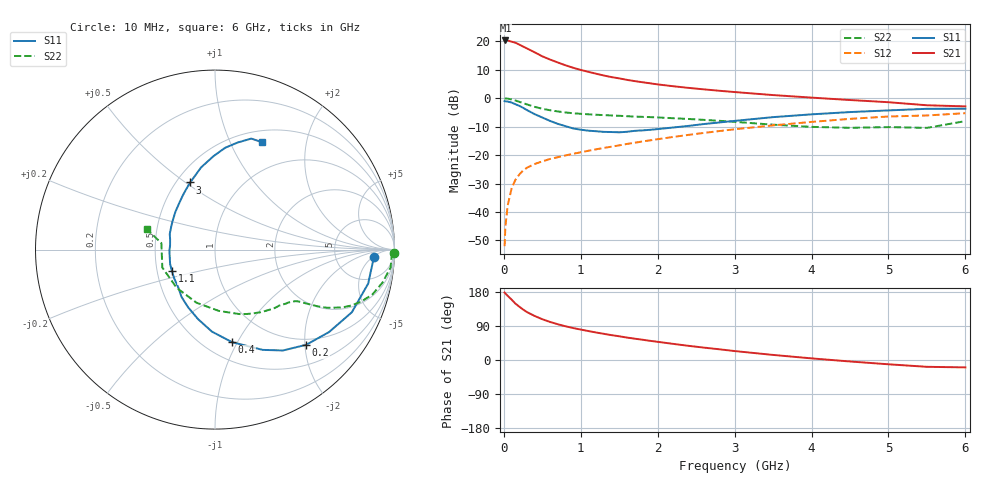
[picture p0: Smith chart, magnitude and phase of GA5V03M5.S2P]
! Infineon Technologies  Discrete & RF Semiconductors
! BF775
! Si NPN RF Bipolar Junction Transistor in SOT23
! VCE = 5 V  IC = 3.5 mA
! Common Emitter S-Parameters:  May  1996
# GHz  S  MA  R  50
!  f  S11  S21  S12  S22
! GHz  MAG  ANG  MAG  ANG  MAG  ANG  MAG  ANG
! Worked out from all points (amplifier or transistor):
!   36 points, 10 MHz to 6 GHz, reference 50 ohm
!   highest |S21| = 20.3 dB at 20 MHz (marker M1)
!   |S21| within 3 dB of that: start of sweep to 315.4 MHz
!   unconditionally stable (mu >= 1): 945.7 MHz to 3.352 GHz
!   at 250 MHz: K = 0.38, MSG = 21.8 dB, |S12| = -25.4 dB
!   at 1.4 GHz: K = 1.12, MAG = 10.2 dB, |S12| = -17.0 dB
!   at 6 GHz: K = 0.95, MSG = 1.2 dB, |S12| = -5.3 dB
!   S11 on the Smith chart (normalised r, x): 10 MHz: 15, -5; 200 MHz: 0.88, -2.03; 400 MHz: 0.67, -0.95; 1.1 GHz: 0.60, -0.15; 3 GHz: 0.59, +0.52; 6 GHz: 0.64, +1.33
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0.01  0.8876 -2.5  10.25 177.9  0.0025 86.6  0.9951 -1.1
0.02  0.8812 -5.0  10.36 175.5  0.0055 85.3  0.9848 -2.2
0.05  0.8742 -12.5  10.33 169.3  0.013 84.0  0.9832 -5.8
0.1  0.8386 -24.6  9.869 159.5  0.0256 76.8  0.9516 -11.1
0.15  0.784 -35.9  9.449 148.9  0.0366 70.3  0.9121 -15.9
0.2  0.7345 -46.2  8.785 140.9  0.0454 66.2  0.8656 -19.5
0.25  0.6779 -56.0  8.1 133.3  0.0534 62.2  0.8209 -22.3
0.3  0.6185 -64.6  7.516 126.5  0.0599 59.9  0.7778 -24.5
0.4  0.5242 -79.6  6.416 116.3  0.0696 55.7  0.7045 -27.4
0.5  0.4575 -92.1  5.45 107.6  0.0775 53.7  0.651 -29.0
0.6  0.3987 -103.7  4.788 100.5  0.0853 52.7  0.6144 -29.9
0.7  0.3546 -115.0  4.256 94.4  0.0916 52.7  0.5855 -30.7
0.9  0.2942 -133.9  3.432 84.4  0.1052 53.1  0.5438 -32.0
1.1  0.2683 -153.7  2.904 76.4  0.1191 53.8  0.5211 -33.8
1.3  0.2557 -170.5  2.505 69.1  0.1336 54.0  0.5037 -35.9
1.6  0.2567 167.0  2.102 59.2  0.1569 54.4  0.4825 -39.7
2.2  0.3052 136.2  1.624 42.6  0.2081 53.0  0.4447 -49.9
3  0.399 110.2  1.283 23.6  0.2842 47.3  0.384 -69.3
3.5  0.4646 99.6  1.135 13.4  0.3329 42.3  0.3422 -86.4
4.5  0.5702 84.3  0.929 -3.9  0.433 30.1  0.3016 -135.1
5.5  0.6508 71.9  0.751 -18.0  0.4969 14.6  0.3008 173.1
6  0.6531 66.3  0.718 -19.5  0.5457 10.3  0.3957 163.4
